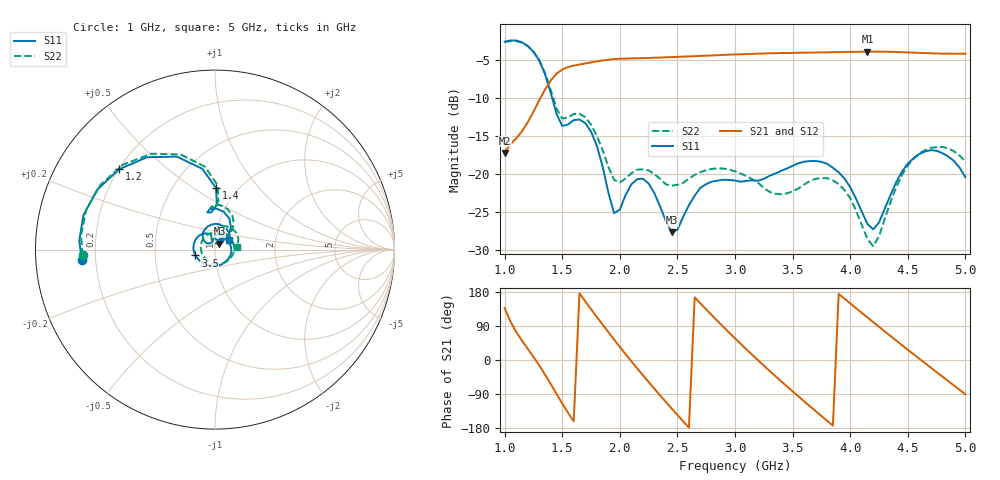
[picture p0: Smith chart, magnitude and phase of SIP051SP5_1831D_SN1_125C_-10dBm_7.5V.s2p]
# GHz  S  dB  R  50
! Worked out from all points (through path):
!   81 points, 1 GHz to 5 GHz, reference 50 ohm
!   highest |S21| = -3.88 dB at 4.15 GHz (marker M1); lowest = -17.2 dB at 1 GHz (marker M2)
!   lowest |S11| = -27.6 dB at 2.45 GHz (marker M3), VSWR 1.09, Z = 52.4 + j3.49 ohm
!   |S11| at or under -10 dB: 1.413 GHz to end of sweep
!   |S22| runs from -29.5 to -2.5 dB; largest |S21 - S12| = 0.0028
!   S11 on the Smith chart (normalised r, x): 1 GHz: 0.15, -0.04; 1.2 GHz: 0.20, +0.35; 1.4 GHz: 0.80, +0.62; 3.5 GHz: 0.80, -0.05; 5 GHz: 1.16, +0.13
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1  -2.57 -175.5  -17.19 137.2  -17.20 137.3  -2.63 -177.5
1.2  -3.13 140.1  -13.20 29.9  -13.20 29.9  -3.13 137.2
1.4  -9.27 89.1  -7.69 -63.3  -7.67 -63.2  -8.93 87.6
1.5  -13.66 96.0  -6.24 -114.6  -6.23 -114.6  -12.69 92.2
1.7  -13.29 77.0  -5.43 154.9  -5.43 154.9  -12.51 73.0
1.85  -18.94 46.8  -5.04 93.7  -5.04 93.8  -16.80 48.7
1.95  -25.13 63.4  -4.86 54.1  -4.88 54.1  -20.74 55.4
2.05  -22.76 92.1  -4.80 15.5  -4.81 15.6  -20.56 70.1
2.2  -20.59 68.0  -4.72 -40.0  -4.73 -40.0  -19.37 60.2
2.35  -24.25 44.4  -4.66 -93.5  -4.63 -93.5  -20.62 48.5
2.45  -27.64 53.2  -4.60 -128.0  -4.58 -128.0  -21.52 48.4
2.7  -21.79 48.3  -4.44 149.3  -4.44 149.3  -19.73 37.9
2.85  -20.85 7.4  -4.35 102.3  -4.35 102.3  -19.25 16.3
3  -20.84 -36.7  -4.25 57.1  -4.26 57.1  -19.62 -11.4
3.25  -20.62 -107.5  -4.12 -14.8  -4.12 -14.8  -21.81 -76.2
3.5  -18.91 -163.5  -4.05 -82.8  -4.04 -82.8  -22.27 -171.2
3.7  -18.26 155.0  -4.00 -134.9  -3.99 -134.9  -20.61 124.2
3.9  -19.75 118.1  -3.94 174.4  -3.93 174.4  -21.31 77.5
4.15  -26.56 107.6  -3.88 112.3  -3.87 112.3  -28.53 61.0
4.35  -22.74 141.9  -3.90 63.3  -3.92 63.3  -23.66 108.5
4.65  -17.03 97.3  -4.07 -8.3  -4.08 -8.4  -16.85 64.9
5  -20.40 34.4  -4.16 -90.5  -4.17 -90.6  -18.32 8.2
